|-- THIS SOFTWARE IS PROVIDED BY FREESCALE "AS IS" AND ANY EXPRESSED OR
|-- IMPLIED WARRANTIES, INCLUDING, BUT NOT LIMITED TO, THE IMPLIED WARRANTIES
|-- OF MERCHANTABILITY AND FITNESS FOR A PARTICULAR PURPOSE ARE DISCLAIMED.
|-- IN NO EVENT SHALL FREESCALE OR ITS CONTRIBUTORS BE LIABLE FOR ANY DIRECT,
|-- INDIRECT, INCIDENTAL, SPECIAL, EXEMPLARY, OR CONSEQUENTIAL DAMAGES
|-- (INCLUDING, BUT NOT LIMITED TO, PROCUREMENT OF SUBSTITUTE GOODS OR
|-- SERVICES; LOSS OF USE, DATA, OR PROFITS; OR BUSINESS INTERRUPTION)
|-- HOWEVER CAUSED AND ON ANY THEORY OF LIABILITY, WHETHER IN CONTRACT,
|-- STRICT LIABILITY, OR TORT (INCLUDING NEGLIGENCE OR OTHERWISE) ARISING
|-- IN ANY WAY OUT OF THE USE OF THIS SOFTWARE, EVEN IF ADVISED OF
|-- THE POSSIBILITY OF SUCH DAMAGE.
[IBIS Ver]   5.0
[Comment Char] |_char
[File name]   k70_120_256mbga_full.ibs
[File Rev]   1.3
[Date]   12/3/2013
[Source]   Freescale, MSG, MCD, Design
[Notes]   IBIS model for K70 microprocessor covers 1.71 - 3.6V range
[Disclaimer]   The model given below represents 256MBGA package on K70 family
[Copyright]   Copyright, Freescale, Inc., 2013
|  Component K70
[Component]   K70
[Manufacturer]  Freescale, Inc.
[Package]
|   typ   min   max
R_pkg   0.18052   0.045308   0.32928
L_pkg   3.318e-9   8.845e-10   6.245e-9
C_pkg   1.59e-12   1.009e-12   2.263e-12
[Pin]   Signal_name   model_name   R_pin   L_pin   C_pin
B1   DDR_VDD   POWER
B5   DDR_VDD   POWER
B8   DDR_VDD   POWER
B12   DDR_VDD   POWER
C16   DDR_VDD   POWER
D2   DDR_VDD   POWER
D4   DDR_VDD   POWER
D7   DDR_VDD   POWER
E10   DDR_VDD   POWER
E12   DDR_VDD   POWER
C6   DDR_VREF   POWER
G7   VDD   POWER
G8   VDD   POWER
G9   VDD   POWER
G10   VDD   POWER
J7   VDD   POWER
J10   VDD   POWER
K10   VDD   POWER
L10   VDD   POWER
N5   VDDA   POWER
H7   VDDINT   POWER
H10   VDDINT   POWER
N3   ADC0SE16   NC   0.13881   2.549e-9   1.57e-12
P3   ADC1SE16   NC   0.17224   2.995e-9   1.722e-12
R3   DAC0OUT   NC   0.22791   4.549e-9   1.671e-12
R4   DAC1OUT   NC   0.21437   4.3e-9   1.531e-12
D10   DDR_A0   pad_st_acc   0.20969   3.108e-9   1.563e-12
C11   DDR_A1   pad_st_acc   0.28723   5.482e-9   1.633e-12
B11   DDR_A2   pad_st_acc   0.22789   3.859e-9   1.52e-12
C12   DDR_A3   pad_st_acc   0.29257   4.964e-9   1.966e-12
C10   DDR_A4   pad_st_acc   0.20313   3.198e-9   1.273e-12
A13   DDR_A5   pad_st_acc   0.2709   4.856e-9   1.479e-12
A14   DDR_A6   pad_st_acc   0.29687   5.28e-9   1.551e-12
D11   DDR_A7   pad_st_acc   0.24885   4.468e-9   1.899e-12
A15   DDR_A8   pad_st_acc   0.30942   5.28e-9   1.735e-12
B15   DDR_A9   pad_st_acc   0.28364   4.791e-9   2.086e-12
B13   DDR_A10   pad_st_acc   0.23743   4.014e-9   1.552e-12
B14   DDR_A11   pad_st_acc   0.24107   3.997e-9   1.908e-12
C15   DDR_A12   pad_st_acc   0.28358   4.488e-9   1.974e-12
D16   DDR_A13   pad_st_acc   0.28942   4.801e-9   1.932e-12
D15   DDR_A14   pad_st_acc   0.28023   4.758e-9   1.957e-12
A9   DDR_BA0   pad_st_acc   0.27029   4.394e-9   1.346e-12
B10   DDR_BA1   pad_st_acc   0.27129   5.131e-9   1.44e-12
B9   DDR_BA2   pad_st_acc   0.22714   3.921e-9   1.447e-12
C13   DDR_CAS_B   pad_st_acc   0.22224   3.203e-9   1.766e-12
A11   DDR_CK   pad_st_clk   0.27682   4.389e-9   1.383e-12
A10   DDR_CKB   pad_st_clk   0.26897   4.548e-9   1.404e-12
B16   DDR_CKE   pad_st_acc   0.31202   4.953e-9   2.13e-12
D14   DDR_CS_B   pad_st_acc   0.24987   4.099e-9   1.719e-12
D9   DDR_DM0   pad_st_dq   0.24692   3.884e-9   1.628e-12
A3   DDR_DM1   pad_st_dq   0.26547   4.507e-9   1.724e-12
C5   DDR_DQ0   pad_st_dq   0.22017   3.658e-9   1.701e-12
B4   DDR_DQ1   pad_st_dq   0.2522   4.497e-9   1.559e-12
A4   DDR_DQ2   pad_st_dq   0.27608   4.635e-9   1.764e-12
B6   DDR_DQ3   pad_st_dq   0.23959   3.865e-9   1.561e-12
D6   DDR_DQ4   pad_st_dq   0.23611   3.99e-9   1.7e-12
A6   DDR_DQ5   pad_st_dq   0.23294   3.874e-9   1.458e-12
B7   DDR_DQ6   pad_st_dq   0.23122   3.27e-9   1.449e-12
A8   DDR_DQ7   pad_st_dq   0.25089   4.164e-9   1.302e-12
D1   DDR_DQ8   pad_st_dq   0.27187   4.728e-9   1.47e-12
C1   DDR_DQ9   pad_st_dq   0.26914   4.26e-9   1.496e-12
C2   DDR_DQ10   pad_st_dq   0.26808   4.412e-9   1.725e-12
B2   DDR_DQ11   pad_st_dq   0.24691   4.185e-9   1.809e-12
C3   DDR_DQ12   pad_st_dq   0.24688   3.776e-9   1.66e-12
C4   DDR_DQ13   pad_st_dq   0.23625   3.428e-9   1.803e-12
B3   DDR_DQ14   pad_st_dq   0.24465   4.025e-9   1.701e-12
A2   DDR_DQ15   pad_st_dq   0.27352   4.654e-9   1.664e-12
C8   DDR_DQS0   pad_st_dqs   0.19294   3.186e-9   1.423e-12
D3   DDR_DQS1   pad_st_dqs   0.21331   2.93e-9   1.559e-12
A7   DDR_ODT   pad_st_acc   0.22028   3.517e-9   1.394e-12
E16   DDR_RAS_B   pad_st_acc   0.32928   5.547e-9   1.686e-12
D13   DDR_WE_B   pad_st_acc   0.20363   3.269e-9   1.748e-12
T5   EXTAL32   NC   0.19859   3.663e-9   1.605e-12
R2   PGA0DM   NC   0.27053   5.572e-9   2.035e-12
R1   PGA0DP   NC   0.27352   5.659e-9   1.95e-12
T2   PGA1DM   NC   0.30594   6.089e-9   1.974e-12
T1   PGA1DP   NC   0.30674   6.245e-9   2.023e-12
N2   PGA2DM   NC   0.23561   4.805e-9   1.494e-12
N1   PGA2DP   NC   0.249   5.08e-9   1.48e-12
P2   PGA3DM   NC   0.25092   5.179e-9   1.872e-12
P1   PGA3DP   NC   0.25763   5.345e-9   1.873e-12
T7   PTA0   io_5vtol   0.16747   3.147e-9   1.524e-12
N8   PTA1   io_5vtol   0.10538   1.879e-9   1.563e-12
T8   PTA2   io_5vtol   0.19012   3.578e-9   1.27e-12
P8   PTA3   io_5vtol   0.13468   2.474e-9   1.376e-12
R8   PTA4   io_5vtol   0.16318   2.999e-9   1.545e-12
T12   PTA5   io_5vtol   0.24941   5.623e-9   1.462e-12
R12   PTA6   io_fast_5vtol   0.20222   4.321e-9   1.749e-12
P12   PTA7   io_fast_5vtol   0.19858   4.208e-9   1.791e-12
N12   PTA8   io_fast_5vtol   0.17789   3.757e-9   2.161e-12
T13   PTA9   io_fast_5vtol   0.24037   4.968e-9   1.563e-12
P13   PTA10   io_fast_5vtol   0.17939   3.758e-9   2.009e-12
R13   PTA11   io_fast_5vtol   0.18669   3.991e-9   1.893e-12
M10   PTA12   io_fast_5vtol   0.11263   2.053e-9   1.26e-12
N10   PTA13   io_fast_5vtol   0.13007   2.381e-9   1.481e-12
R11   PTA14   io_fast_5vtol   0.16577   3.04e-9   1.255e-12
P11   PTA15   io_fast_5vtol   0.14338   2.554e-9   1.187e-12
N11   PTA16   io_fast_5vtol   0.1217   2.186e-9   1.14e-12
T11   PTA17   io_fast_5vtol   0.19461   3.614e-9   1.084e-12
T15   PTA18   io_5vtol   0.19376   3.577e-9   1.8e-12
T16   PTA19   io_5vtol   0.20602   3.917e-9   1.743e-12
N13   PTA24   io_fast_5vtol   0.12779   2.505e-9   1.408e-12
R14   PTA25   io_fast_5vtol   0.17389   3.27e-9   1.698e-12
M13   PTA26   io_fast_5vtol   0.113   2.127e-9   1.163e-12
R15   PTA27   io_fast_5vtol   0.18609   3.52e-9   1.668e-12
P14   PTA28   io_fast_5vtol   0.16516   3.161e-9   1.82e-12
N14   PTA29   io_fast_5vtol   0.15954   3.051e-9   1.456e-12
M12   PTB0   io_5vtol   0.13454   2.548e-9   1.611e-12
M11   PTB1   io_5vtol   0.15085   2.852e-9   1.633e-12
P15   PTB2   io_5vtol   0.19504   3.845e-9   1.704e-12
M14   PTB3   io_5vtol   0.15299   3.03e-9   1.872e-12
N15   PTB4   io_5vtol   0.17742   3.428e-9   1.709e-12
M15   PTB5   io_5vtol   0.1751   3.373e-9   1.558e-12
L14   PTB6   io_5vtol   0.13653   2.621e-9   2.027e-12
L15   PTB7   io_5vtol   0.16591   3.319e-9   1.927e-12
K14   PTB8   io_5vtol   0.13096   2.505e-9   1.902e-12
K15   PTB9   io_5vtol   0.14021   2.769e-9   1.07e-12
J13   PTB10   io_5vtol   0.09459   1.76e-9   1.855e-12
J14   PTB11   io_5vtol   0.12514   2.593e-9   1.816e-12
J15   PTB16   io_5vtol   0.15453   3.087e-9   1.653e-12
H13   PTB17   io_5vtol   0.092563   1.739e-9   1.636e-12
H14   PTB18   io_5vtol   0.12313   2.468e-9   1.637e-12
H15   PTB19   io_5vtol   0.14382   2.854e-9   1.597e-12
G13   PTB20   io_5vtol   0.10269   1.86e-9   1.16e-12
G14   PTB21   io_5vtol   0.12654   2.485e-9   1.539e-12
G15   PTB22   io_5vtol   0.15548   2.97e-9   1.608e-12
H16   PTB23   io_5vtol   0.19783   4.064e-9   1.41e-12
G16   PTC0   io_5vtol   0.18526   3.579e-9   1.386e-12
F13   PTC1   io_5vtol   0.10401   1.942e-9   1.589e-12
F14   PTC2   io_5vtol   0.13142   2.476e-9   1.539e-12
E13   PTC3   io_5vtol   0.1004   1.957e-9   1.663e-12
E14   PTC4   io_5vtol   0.11994   2.299e-9   1.489e-12
E15   PTC5   io_5vtol   0.15686   2.928e-9   1.584e-12
F12   PTC6   io_5vtol   0.078755   1.4e-9   1.438e-12
G12   PTC7   io_5vtol   0.11949   2.138e-9   1.234e-12
H12   PTC8   io_5vtol   0.12243   2.364e-9   1.725e-12
F11   PTC9   io_5vtol   0.10337   1.725e-9   1.41e-12
G11   PTC10   io_5vtol   0.10449   1.798e-9   1.607e-12
H11   PTC11   io_5vtol   0.11345   1.971e-9   1.461e-12
J12   PTC12   io_5vtol   0.16597   3.006e-9   1.995e-12
K13   PTC13   io_5vtol   0.18035   3.386e-9   1.85e-12
J11   PTC14   io_5vtol   0.15476   2.9e-9   2.063e-12
F10   PTC15   io_5vtol   0.077802   1.316e-9   1.763e-12
F9   PTC16   io_5vtol   0.11546   2.104e-9   1.71e-12
E9   PTC17   io_5vtol   0.073418   1.222e-9   1.199e-12
M9   PTC18   io_5vtol   0.20103   3.697e-9   1.934e-12
M8   PTC19   io_5vtol   0.21304   3.921e-9   1.964e-12
L8   PTD0   io_5vtol   0.18575   3.348e-9   2.263e-12
F8   PTD1   io_5vtol   0.093904   1.575e-9   1.203e-12
K6   PTD2   io_5vtol   0.17646   3.227e-9   2.206e-12
J6   PTD3   io_5vtol   0.1608   2.954e-9   1.975e-12
K5   PTD4   io_5vtol   0.20746   3.794e-9   2.002e-12
J5   PTD5   io_5vtol   0.16794   3.071e-9   2.138e-12
K4   PTD6   io_5vtol   0.24544   4.399e-9   1.751e-12
E7   PTD7   io_5vtol   0.045308   8.845e-10   1.269e-12
J4   PTD8   io_5vtol   0.14803   2.926e-9   1.866e-12
F7   PTD9   io_5vtol   0.082935   1.407e-9   1.176e-12
E6   PTD10   io_5vtol   0.076184   1.168e-9   1.009e-12
G5   PTD11   io_5vtol   0.11621   2.062e-9   1.707e-12
F5   PTD12   io_5vtol   0.091187   1.514e-9   1.162e-12
F4   PTD13   io_5vtol   0.12   2.129e-9   1.16e-12
E5   PTD14   io_5vtol   0.098071   1.744e-9   1.155e-12
E4   PTD15   io_5vtol   0.11233   1.961e-9   1.231e-12
E2   PTE0   io_5vtol   0.14813   2.822e-9   1.514e-12
F2   PTE1   io_5vtol   0.16956   3.254e-9   1.727e-12
F3   PTE2   io_5vtol   0.11926   2.243e-9   1.577e-12
G2   PTE3   io_5vtol   0.15207   2.885e-9   1.616e-12
G3   PTE4   io_5vtol   0.12576   2.367e-9   1.503e-12
G4   PTE5   io_5vtol   0.12367   2.279e-9   1.433e-12
H2   PTE6   io_5vtol   0.14867   2.849e-9   1.445e-12
H3   PTE7   io_5vtol   0.13493   2.545e-9   1.493e-12
H4   PTE8   io_5vtol   0.12145   2.262e-9   1.485e-12
J1   PTE9   io_5vtol   0.19253   3.912e-9   1.311e-12
J2   PTE10   io_5vtol   0.15509   2.915e-9   1.579e-12
K1   PTE11   io_5vtol   0.20312   3.806e-9   1.435e-12
K3   PTE12   io_5vtol   0.16058   3.242e-9   1.628e-12
J3   PTE16   io_5vtol   0.1239   2.263e-9   1.545e-12
K2   PTE17   io_5vtol   0.15961   2.895e-9   1.578e-12
L4   PTE18   io_5vtol   0.13369   2.686e-9   1.569e-12
M3   PTE19   io_5vtol   0.23888   4.797e-9   1.85e-12
P7   PTE24   io_5vtol   0.14027   2.492e-9   1.268e-12
R7   PTE25   io_5vtol   0.14281   2.607e-9   1.314e-12
M7   PTE26   io_5vtol   0.070296   1.237e-9   1.21e-12
K7   PTE27   io_5vtol   0.074541   1.376e-9   1.545e-12
L7   PTE28   io_5vtol   0.094016   1.697e-9   1.455e-12
P16   PTF0   io_5vtol   0.20391   4.004e-9   1.503e-12
L13   PTF1   io_5vtol   0.11616   2.163e-9   1.121e-12
N16   PTF2   io_5vtol   0.23074   4.401e-9   1.741e-12
M16   PTF3   io_5vtol   0.22239   4.261e-9   1.69e-12
L16   PTF4   io_5vtol   0.20336   3.961e-9   1.602e-12
K16   PTF5   io_5vtol   0.1956   3.795e-9   1.447e-12
J16   PTF6   io_5vtol   0.18851   3.626e-9   1.455e-12
F15   PTF7   io_5vtol   0.15643   2.914e-9   1.496e-12
F16   PTF8   io_5vtol   0.17864   3.631e-9   1.392e-12
K12   PTF9   io_5vtol   0.17116   3.183e-9   2.099e-12
L12   PTF10   io_5vtol   0.2029   3.721e-9   1.972e-12
K11   PTF11   io_5vtol   0.19338   3.438e-9   2.186e-12
L11   PTF12   io_5vtol   0.20971   3.733e-9   2.186e-12
H6   PTF13   io_5vtol   0.17111   2.917e-9   1.872e-12
G6   PTF14   io_5vtol   0.12516   2.183e-9   1.551e-12
F6   PTF15   io_5vtol   0.084644   1.476e-9   1.065e-12
E1   PTF16   io_5vtol   0.18109   3.872e-9   1.359e-12
F1   PTF17   io_5vtol   0.19574   3.933e-9   1.33e-12
G1   PTF18   io_5vtol   0.19077   3.618e-9   1.264e-12
H1   PTF19   io_5vtol   0.18666   3.579e-9   1.272e-12
H5   PTF20   io_5vtol   0.11851   2.214e-9   1.019e-12
P9   PTF21   io_5vtol   0.12022   2.137e-9   1.423e-12
N9   PTF22   io_5vtol   0.10331   1.836e-9   1.344e-12
P10   PTF23   io_fast_5vtol   0.12233   2.285e-9   1.551e-12
R10   PTF24   io_fast_5vtol   0.19087   3.953e-9   1.44e-12
R9   PTF25   io_fast_5vtol   0.21369   4.417e-9   1.666e-12
T9   PTF26   io_fast_5vtol   0.24827   5.309e-9   1.654e-12
T10   PTF27   io_fast_5vtol   0.24201   4.734e-9   1.438e-12
R16   RESETB   io_3v   0.13636   3.36e-9   2.068e-12
M5   RTC_WAKEUP_B   io_3v   0.09656   1.873e-9   1.488e-12
L5   TAMPER1   io_3v   0.12068   2.21e-9   1.314e-12
L6   TAMPER2   io_3v_trig   0.10977   2.162e-9   1.761e-12
R5   TAMPER3   io_3v   0.20495   4.242e-9   1.62e-12
P6   TAMPER4   io_3v   0.18943   4.019e-9   1.479e-12
R6   TAMPER5   io_3v_trig   0.19377   3.913e-9   1.309e-12
N6   TAMPER6   io_3v_trig   0.078755   1.388e-9   1.022e-12
M6   TAMPER7   io_3v   0.061931   1.078e-9   1.365e-12
M2   USB0DM   NC   0.21249   3.802e-9   1.521e-12
M1   USB0DP   NC   0.22419   3.937e-9   1.626e-12
P5   VBAT   POWER   0.086743   2.279e-9   1.473e-12
L1   VOUT33   POWER   0.1084   2.372e-9   1.413e-12
P4   VREFH   NC   0.22007   4.158e-9   1.683e-12
M4   VREFL   NC   0.1706   3.057e-9   1.722e-12
T3   VREFOUT   NC   0.25241   5.095e-9   1.381e-12
L3   VREGIN   POWER   0.093829   2.12e-9   1.221e-12
T6   XTAL32   NC   0.19157   3.587e-9   1.515e-12
A1   DDR_VSS   GND
A5   DDR_VSS   GND
A12   DDR_VSS   GND
A16   DDR_VSS   GND
C7   DDR_VSS   GND
C9   DDR_VSS   GND
C14   DDR_VSS   GND
D8   DDR_VSS   GND
D12   DDR_VSS   GND
E3   DDR_VSS   GND
D5   DDR_VSS_BULK   GND
E8   DDR_VSS_BULK   GND
E11   DDR_VSS_BULK   GND
H8   VSS   GND
H9   VSS   GND
J8   VSS   GND
J9   VSS   GND
K8   VSS   GND
K9   VSS   GND
L2   VSS   GND
L9   VSS   GND
N7   VSS   GND
T4   VSS   GND
T14   VSS   GND
N4   VSSA   GND
[Diff Pin] inv_pin vdiff tdelay_typ tdelay_min tdelay_max
A11 A10   NA   NA   NA   NA | Output* pin pair
|End [Component]
[Component] io65u65dgo6m3v
|   Component io65u65dgo6m3v
| This component was characterised for following simulation conditions:
| Temperature:
|   - Typ: 25.0C,   - Min: 125.0C,   - Max: -40.0C
| External (pad) voltage:
|   - Typ: 3.3V,   - Min: 1.71V,   - Max: 3.6V
| Internal (core) voltage:
|   - Typ: 3.3V,   - Min: 1.71V,   - Max: 3.6V
[Manufacturer] Freescale Semiconductor
[Package]
| variable   typ   min   max
R_pkg   0.2240   0.2240   0.2240
L_pkg   8.5100nH   8.5100nH   8.5100nH
C_pkg   0.2740pF   0.2740pF   0.2740pF
[Pin]  signal_name   model_name   R_pin   L_pin   C_pin
fpad   pad   io_3v_trig
pad   pad   io_3v
vdd3v  vdd3v   POWER
vss3v  vss3v   GND
|obe   obe   dummy
|do   do   dummy
[Model Selector] io_3v_trig
io_3v_trig_dse1_sre0   io with trigger, full drive mode without slew rate
io_3v_trig_dse1_sre1   io with trigger, full drive mode with slew rate
io_3v_trig_dse0_sre0   io with trigger, low drive mode without slew rate
io_3v_trig_dse0_sre1   io with trigger, low drive mode with slew rate
[Model Selector] io_3v
io_3v_dse1_sre0   io, full drive mode without slew rate
io_3v_dse1_sre1   io, full drive mode with slew rate
io_3v_dse0_sre0   io, low drive mode without slew rate
io_3v_dse0_sre1   io, low drive mode with slew rate
[Component] io80u65dgo6m5vtol
|   Component io80u65dgo6m5vtol
| This component was characterised for following simulation conditions:
| Spice Models:
|  - Typ Condition
|   /proj/tec16/analog/modules/IO_C90/io80u65dgo4m5vtol/users/antony/ibis/io80u/6m1t/cmos090sgtfs_typ.model
|  - Min Condition
|   /proj/tec16/analog/modules/IO_C90/io80u65dgo4m5vtol/users/antony/ibis/io80u/6m1t/cmos090sgtfs_wcs.model
|  - Max Condition
|   /proj/tec16/analog/modules/IO_C90/io80u65dgo4m5vtol/users/antony/ibis/io80u/6m1t/cmos090sgtfs_bcs.model
| Spice  Netlist:
|  - Typ Condition
|   /proj/tec16/analog/modules/IO_C90/io80u65dgo4m5vtol/users/antony/ibis/io80u/6m1t/io.ckt
|  - Min Condition
|   /proj/tec16/analog/modules/IO_C90/io80u65dgo4m5vtol/users/antony/ibis/io80u/6m1t/io.ckt
|  - Max Condition
|   /proj/tec16/analog/modules/IO_C90/io80u65dgo4m5vtol/users/antony/ibis/io80u/6m1t/io.ckt
| Temperature:
|   - Typ: 25.0C,   - Min: 125.0C,   - Max: -40.0C
| External (pad) voltage:
|   - Typ: 3.3V,   - Min: 1.71V,   - Max: 3.6V
| Internal (core) voltage:
|   - Typ: 1.2V,   - Min: 1.08V,   - Max: 1.32V
[Manufacturer] Freescale Semiconductor
[Package]
| variable   typ   min   max
R_pkg   0.2240   0.2240   0.2240
L_pkg   8.5100nH   8.5100nH   8.5100nH
C_pkg   0.2740pF   0.2740pF   0.2740pF
[Pin]  signal_name   model_name   R_pin   L_pin   C_pin
fpad   pad   io_fast_5vtol
pad   pad   io_5vtol
|vsslv vsslv   iGND
|vddlv vddlv   iPOWER
vdd3v  vdd3v   POWER
vss3v  vss3v   GND
|obe   obe   dummy
|do   do   dummy
[Model Selector] io_fast_5vtol
io_fast_5vtol_dse1_sre0   fast io, full drive mode without slew rate
io_fast_5vtol_dse1_sre1   fast io, full drive mode with slew rate
io_fast_5vtol_dse0_sre0   fast io, low drive mode without slew rate
io_fast_5vtol_dse0_sre1   fast io, low drive mode with slew rate
[Model Selector] io_5vtol
io_5vtol_dse1_sre0   io, full drive mode without slew rate
io_5vtol_dse1_sre1   io, full drive mode with slew rate
io_5vtol_dse0_sre0   io, low drive mode without slew rate
io_5vtol_dse0_sre1   io, low drive mode with slew rate
|   Component pad_st_acc
[Component]   pad_st_acc
[Manufacturer]   Freescale Semiconductor
[Package]
| variable  typ   min   max
R_pkg   2.24E-01   2.24E-01   2.24E-01
L_pkg   8.51E-09   8.51E-09   8.51E-09
C_pkg   0.27E-12   0.27E-12   0.27E-12
[Pin]  signal_name   model_name   R_pin   L_pin   C_pin
| in   in   dummy
| obe  obe   dummy
vsse   vsse   GND
vdde   vdde   POWER
pad   pad   pad_st_acc
|   Model Selector
[Model Selector] pad_st_acc
| 1.8V VDDE
ac18_000  LPDDR Half Strength
ac18_001  LPDDR Full Strength
ac18_010  DDR2 Half Strength
ac18_110  DDR2 Full Strength
| 2.5V VDDE
ac25_011  DDR1
|   Component pad_st_clk
[Component]   pad_st_clk
[Manufacturer]   Freescale Semiconductor
[Package]
| variable  typ   min   max
R_pkg   2.24E-01   2.24E-01   2.24E-01
L_pkg   8.51E-09   8.51E-09   8.51E-09
C_pkg   0.27E-12   0.27E-12   0.27E-12
[Pin]  signal_name   model_name   R_pin   L_pin   C_pin
| in   in   dummy
| obe  obe   dummy
vsse   vsse   GND
vdde   vdde   POWER
pad   pad   pad_st_clk
|   Model Selector
[Model Selector] pad_st_clk
| 1.8V VDDE
ck18_000  LPDDR Half Strength
ck18_001  LPDDR Full Strength
ck18_010  DDR2 Half Strength
ck18_110  DDR2 Full Strength
| 2.5V VDDE
ck25_011  DDR1
|   Component pad_st_dq
[Component]   pad_st_dq
[Manufacturer]   Freescale Semiconductor
[Package]
| variable  typ   min   max
R_pkg   2.24E-01   2.24E-01   2.24E-01
L_pkg   8.51E-09   8.51E-09   8.51E-09
C_pkg   0.27E-12   0.27E-12   0.27E-12
[Pin]  signal_name   model_name   R_pin   L_pin   C_pin
| in   in   dummy
| obe  obe   dummy
vsse   vsse   GND
vdde   vdde   POWER
pad   pad   pad_st_dq
|   Model Selector
[Model Selector] pad_st_dq
| 1.8V VDDE
dq18_000  LPDDR Half Strength
dq18_001  LPDDR Full Strength
dq18_010  DDR2 Half Strength
dq18_110  DDR2 Full Strength
dqin18_000  DDR2 input 1.8V with no termination
dqin18_075  DDR2 input 1.8V with 75 Ohms termination
dqin18_150  DDR2 input 1.8V with 150 Ohms termination
| 2.5V VDDE
dq25_011  DDR1
dqin25_000  DDR1 input 2.5V with no termination
|   Component pad_st_dqs
[Component]   pad_st_dqs
[Manufacturer]   Freescale Semiconductor
[Package]
| variable  typ   min   max
R_pkg   2.24E-01   2.24E-01   2.24E-01
L_pkg   8.51E-09   8.51E-09   8.51E-09
C_pkg   0.27E-12   0.27E-12   0.27E-12
[Pin]  signal_name   model_name   R_pin   L_pin   C_pin
| in   in   dummy
| obe  obe   dummy
vsse   vsse   GND
vdde   vdde   POWER
pad   pad   pad_st_dqs
|   Model Selector
[Model Selector] pad_st_dqs
| 1.8V VDDE
ds18_000  LPDDR Half Strength
ds18_001  LPDDR Full Strength
ds18_010  DDR2 Half Strength
ds18_110  DDR2 Full Strength
dsin18_000  DDR2 input 1.8V with no termination
dsin18_075  DDR2 input 1.8V with 75 Ohms termination
dsin18_150  DDR2 input 1.8V with 150 Ohms termination
| 2.5V VDDE
ds25_011  DDR1
dsin25_000  DDR1 input 2.5V with no termination
| Models and submodels in the file (44): io_3v_trig_dse1_sre0 (I/O), io_3v_dse1_sre0 (I/O), io_3v_trig_dse1_sre1 (I/O), io_3v_dse1_sre1 (I/O), io_3v_trig_dse0_sre0 (I/O), io_3v_dse0_sre0 (I/O), io_3v_trig_dse0_sre1 (I/O), io_3v_dse0_sre1 (I/O), io_fast_5vtol_dse1_sre0 (I/O), io_5vtol_dse1_sre0 (I/O), io_fast_5vtol_dse1_sre1 (I/O), io_5vtol_dse1_sre1 (I/O), io_fast_5vtol_dse0_sre0 (I/O), io_5vtol_dse0_sre0 (I/O), io_fast_5vtol_dse0_sre1 (I/O), io_5vtol_dse0_sre1 (I/O), ac18_000 (Output), ac18_001 (Output), ac18_010 (Output), ac18_110 (Output), ac25_011 (Output), ck18_000 (Output), ck18_001 (Output), ck18_010 (Output), ck18_110 (Output), ck25_011 (Output), dq18_000 (3-state), dq18_001 (3-state), dq18_010 (3-state), dq18_110 (3-state), dqin18_000 (Input), dqin18_075 (Input), dqin18_150 (Input), dq25_011 (3-state), dqin25_000 (Input), ds18_000 (3-state), ds18_001 (3-state), ds18_010 (3-state), ds18_110 (3-state), dsin18_000 (Input), dsin18_075 (Input), dsin18_150 (Input), ds25_011 (3-state), dsin25_000 (Input)
